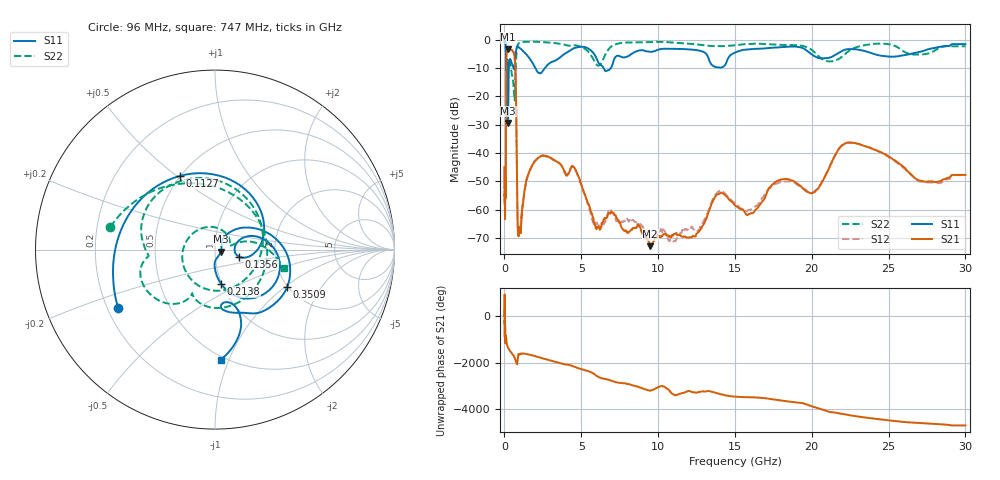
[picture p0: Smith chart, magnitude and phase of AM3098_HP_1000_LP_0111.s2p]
! Date/Time: Thu, Feb 28, 2019 8:39 AM
! Network Analyzer: Agilent Technologies E8364B Rev: A.07.50.67
! Sweep from 0.010 to 30.000 GHz, 1601 Points, Sweep Type: LOG
! Power Supply: 5.023 V, 0.002 A
# Hz S DB R 50
!freq MagS11 AngS11 MagS21 AngS21 MagS12 AngS12 MagS22 AngS22
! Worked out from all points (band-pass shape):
!   1601 points, 10 MHz to 30 GHz, reference 50 ohm
!   highest |S21| = -3.42 dB at 235.1 MHz (marker M1); lowest = -72.8 dB at 9.49 GHz (marker M2)
!   |S21| within 3 dB of the highest: 127.3 MHz to 664.3 MHz (537 MHz wide, 136 % of centre)
!   lowest |S11| = -29.4 dB at 236.3 MHz (marker M3), VSWR 1.07, Z = 53.3 - j1.23 ohm
!   |S11| at or under -10 dB: 198.7 MHz to 286.6 MHz (87.92 MHz wide, 36.2 % of centre); 2.008 GHz to 2.643 GHz (635.3 MHz wide, 27.3 % of centre); 6.45 GHz to 6.932 GHz (482.8 MHz wide, 7.22 % of centre)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
!   |S22| runs from -21.5 to -0.6 dB; largest |S21 - S12| = 0.01
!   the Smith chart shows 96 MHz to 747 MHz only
!   S11 on the Smith chart (normalised r, x): 96 MHz: 0.24, -0.26; 112.7 MHz: 0.50, +0.51; 135.6 MHz: 1.30, -0.10; 213.8 MHz: 0.99, -0.39; 350.9 MHz: 1.98, -1.04; 747 MHz: 0.48, -0.93
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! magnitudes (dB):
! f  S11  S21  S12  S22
! 10 MHz  -0.3  -44.9  -46.1  -0.6
! 38.04 MHz  -0.5  -61.6  -59.9  -0.9
! 96 MHz  -4.0  -41.5  -42.3  -4.5
! 112.7 MHz  -6.8  -16.5  -16.5  -10.6
! 135.6 MHz  -17.2  -5.0  -4.9  -11.2
! 144.7 MHz  -18.5  -4.4  -4.4  -10.5
! 213.8 MHz  -14.2  -3.6  -3.5  -8.1
! 235.1 MHz  -29.3  -3.4  -3.4  -8.6
! 236.3 MHz  -29.4  -3.4  -3.4  -8.6
! 350.9 MHz  -6.9  -3.8  -3.8  -7.3
! 550.5 MHz  -9.4  -4.1  -4.1  -13.8
! 662.4 MHz  -9.5  -6.3  -6.3  -21.5
! 747 MHz  -4.2  -18.3  -18.3  -8.0
! 898.9 MHz  -2.6  -69.0  -68.1  -1.5
! 2.084 GHz  -10.8  -42.3  -42.2  -0.8
! 4.525 GHz  -3.1  -45.1  -45.0  -2.0
! 5.989 GHz  -6.6  -66.8  -65.0  -8.8
! 7.926 GHz  -6.1  -67.3  -62.8  -1.1
! 9.49 GHz  -4.3  -72.8  -70.2  -0.9
! 20 GHz  -5.2  -54.2  -54.0  -3.7
! 22.56 GHz  -3.4  -36.3  -36.4  -3.5
! 30 GHz  -1.6  -47.7  -47.8  -2.4
